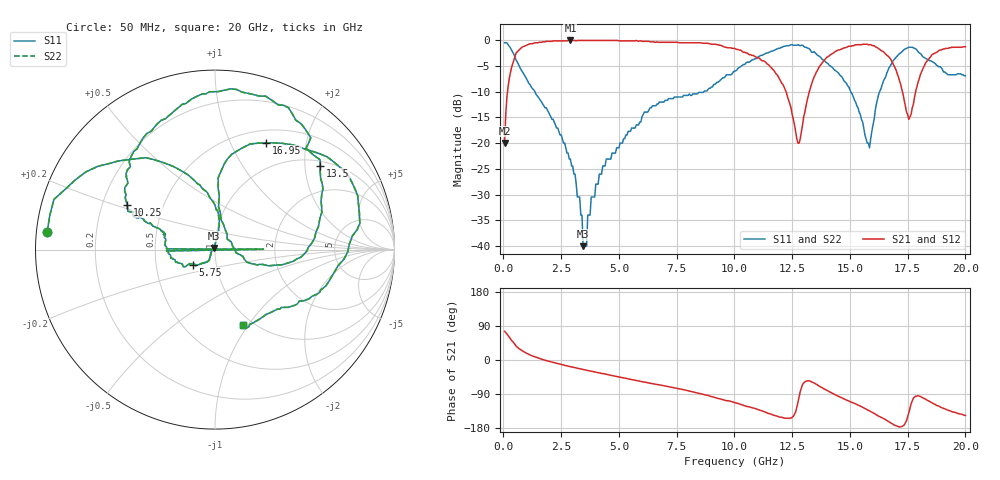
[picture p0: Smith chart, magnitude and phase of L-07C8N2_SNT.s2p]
#	mhz	s	ma	r	50
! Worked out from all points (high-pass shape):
!   400 points, 50 MHz to 20 GHz, reference 50 ohm
!   highest |S21| = -0.09 dB at 2.9 GHz (marker M1); lowest = -20.0 dB at 50 MHz (marker M2)
!   |S21| within 3 dB of the highest: 509.4 MHz to 10.85 GHz (10.34 GHz wide, 182 % of centre); 14.1 GHz to 16.65 GHz (2.543 GHz wide, 16.5 % of centre)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
!   lowest |S11| = -40.0 dB at 3.45 GHz (marker M3), VSWR 1.02, Z = 49.5 + j0.833 ohm
!   |S11| at or under -10 dB: 1.359 GHz to 8.681 GHz (7.322 GHz wide, 146 % of centre); 15.03 GHz to 16.29 GHz (1.257 GHz wide, 8.02 % of centre)
!   |S22| runs from -40.0 to -0.5 dB; largest |S21 - S12| = 0
!   S11 on the Smith chart (normalised r, x): 50 MHz: 0.03, +0.05; 5.75 GHz: 0.77, -0.13; 10.25 GHz: 0.31, +0.22; 13.5 GHz: 1.12, +2.40; 16.95 GHz: 0.65, +1.38; 20 GHz: 0.89, -0.95
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50  0.94 173.9  0.1 75.6  0.1 75.6  0.94 173.9
550  0.64 126.9  0.75 36.5  0.75 36.5  0.64 126.9
2900  0.07 80.2  0.99 -17.6  0.99 -17.6  0.07 80.2
3400  0.02 110.5  0.99 -24.5  0.99 -24.5  0.02 110.5
3450  0.01 122.6  0.99 -25.1  0.99 -25.1  0.01 122.6
4300  0.06 -121.7  0.99 -35.8  0.99 -35.8  0.06 -121.7
5750  0.15 -145.3  0.99 -54.2  0.99 -54.2  0.15 -145.3
6700  0.24 -168.1  0.95 -65.1  0.95 -65.1  0.24 -168.1
7150  0.27 -178.4  0.95 -70.1  0.95 -70.1  0.27 -178.4
7200  0.27 0.4  0.95 -70.8  0.95 -70.8  0.27 0.4
7250  0.27 179.2  0.95 -71.4  0.95 -71.4  0.27 179.2
10050  0.5 155.1  0.82 -113.4  0.82 -113.4  0.5 155.1
10250  0.55 152.9  0.8 -116.9  0.8 -116.9  0.55 152.9
12750  0.9 71.7  0.1 -112.3  0.1 -112.3  0.9 71.7
13350  0.76 48.1  0.38 -58.0  0.38 -58.0  0.76 48.1
13500  0.75 38.6  0.46 -62.3  0.46 -62.3  0.75 38.6
15850  0.09 40.4  0.9 -134.0  0.9 -134.0  0.09 40.4
16700  0.54 79.9  0.68 -163.4  0.68 -163.4  0.54 79.9
16950  0.66 64.3  0.54 -172.5  0.54 -172.5  0.66 64.3
17550  0.85 29.0  0.17 -139.4  0.17 -139.4  0.85 29.0
17950  0.77 5.8  0.39 -94.5  0.39 -94.5  0.77 5.8
20000  0.45 -69.8  0.86 -146.4  0.86 -146.4  0.45 -69.8
